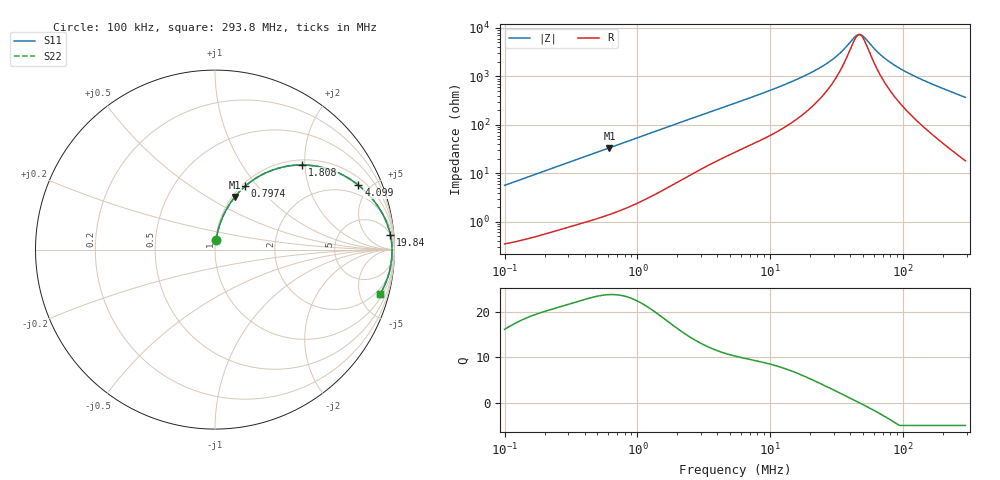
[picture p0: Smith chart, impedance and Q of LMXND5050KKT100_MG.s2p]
! LMXND5050KKT100_MG  S-PARAMETER MODEL  ( General Type )
! Model Generated by TAIYO YUDEN Corporation (http://www.ty-top.com)
! Version 1.0
! TAIYO YUDEN Control No. 191023NI43SB-FBB
! Copyright(c) 2019 TAIYO YUDEN CO.,LTD. All Rights Reserved.
! Product Description (link to TY-COMPAS)
! https://ds.yuden.co.jp/TYCOMPAS/or/detail?pn=LMXND5050KKT100MMG&u=M
! Products Name : Inductors
! Characteristics :
!  Inductance : 10 uH , SRF(min) : 23 MHz , DC Resistance(max) : 0.3 Ohm
!  Rated Current : Saturation :850 mA , Temp Rise : 900 mA
!  Case Size : 4.9 x 4.9 / 0.193 x 0.193 [mm/inch] , Thickness : 1 / 0.039 [mm/inch]
!  (Conditions: Temperature = 25 degC , DC Bias Current/Voltage = 0A / 0V)
! External Node Assignments :
!  1  o---GGG---o  2
! GND o---------o GND
! Frequency Range : 0.1MHz  -  293.796821MHz  [ 402 STEP ]
# MHz S RI R 50
! Freq[MHz].  S11 Real  S11 Imag  S21 Real  S21 Imag  S12 Real  S12 Imag  S22 Real  S22 Imag
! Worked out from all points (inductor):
!   401 points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, 100 kHz to 293.8 MHz, reference 50 ohm
!   read as one part in series: L = 8.92 uH near 104.1 kHz
!   highest Q = 23.8 at 615.1 kHz (marker M1), where L = 8.65 uH
!   self-resonance near 46.7 MHz
!   S11 on the Smith chart (normalised r, x): 100 kHz: 1.01, +0.11; 797.4 kHz: 1.04, +0.86; 1.808 MHz: 1.11, +1.93; 4.099 MHz: 1.38, +4.25; 19.84 MHz: 5, +23; 293.8 MHz: 1.36, -7.34
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0.1  0.00659 0.0557  0.9934 -0.0557  0.9934 -0.0557  0.00659 0.0557
0.205175  0.0183 0.1114  0.9817 -0.1114  0.9817 -0.1114  0.0183 0.1114
0.380976  0.0499 0.1966  0.9501 -0.1966  0.9501 -0.1966  0.0499 0.1966
0.61515  0.1105 0.2932  0.8895 -0.2932  0.8895 -0.2932  0.1105 0.2932
0.797429  0.1677 0.3529  0.8323 -0.3529  0.8323 -0.3529  0.1677 0.3529
1.451429  0.384 0.4611  0.616 -0.4611  0.616 -0.4611  0.384 0.4611
1.807869  0.4842 0.4716  0.5158 -0.4716  0.5158 -0.4716  0.4842 0.4716
2.589579  0.6432 0.4449  0.3568 -0.4449  0.3568 -0.4449  0.6432 0.4449
4.09866  0.7994 0.3587  0.2006 -0.3587  0.2006 -0.3587  0.7994 0.3587
5.420303  0.8637 0.2977  0.1363 -0.2977  0.1363 -0.2977  0.8637 0.2977
11.34535  0.9535 0.1571  0.0465 -0.1571  0.0465 -0.1571  0.9535 0.1571
19.84181  0.9774 0.0816  0.0226 -0.0816  0.0226 -0.0816  0.9774 0.0816
20.65007  0.9783 0.0771  0.0217 -0.0771  0.0217 -0.0771  0.9783 0.0771
30.78391  0.9844 0.0368  0.0156 -0.0368  0.0156 -0.0368  0.9844 0.0368
35.40093  0.9855 0.0241  0.0145 -0.0241  0.0145 -0.0241  0.9855 0.0241
43.22309  0.9863 0.00666  0.0137 -0.00666  0.0137 -0.00666  0.9863 0.00666
45.89085  0.9865 0.0015  0.0135 -0.0015  0.0135 -0.0015  0.9865 0.0015
50.70803  0.9865 -0.0071  0.0135 0.0071  0.0135 0.0071  0.9865 -0.0071
64.43445  0.9859 -0.0282  0.0141 0.0282  0.0141 0.0282  0.9859 -0.0282
78.67184  0.9846 -0.0469  0.0154 0.0469  0.0154 0.0469  0.9846 -0.0469
132.2033  0.9755 -0.1057  0.0245 0.1057  0.0245 0.1057  0.9755 -0.1057
293.7968  0.9206 -0.2468  0.0794 0.2468  0.0794 0.2468  0.9206 -0.2468
